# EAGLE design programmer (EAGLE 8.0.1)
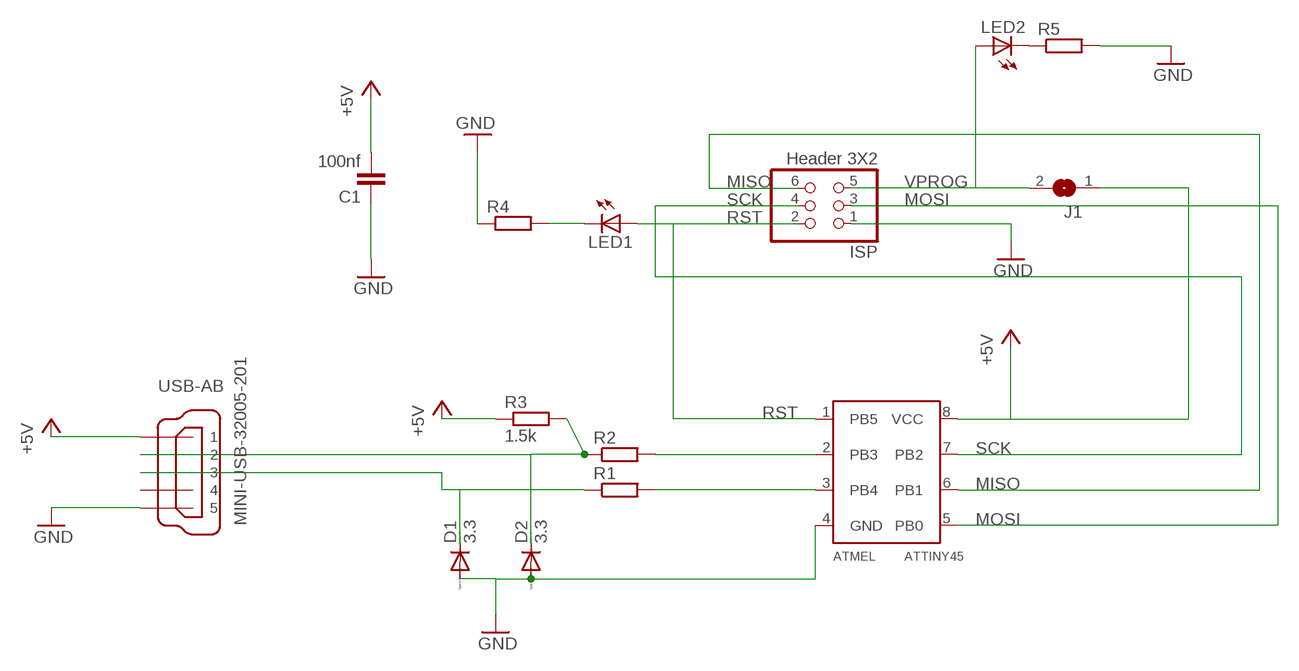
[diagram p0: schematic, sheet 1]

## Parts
ATMEL  ATTINY45  [SOIC8]
C1  100nf  C-EUC1206  [C1206]
D1  3.3  DIODE-MINIMELF  [MINIMELF]
D2  3.3  DIODE-MINIMELF  [MINIMELF]
ISP  Header 3X2  PINHD-2X3SMT  [2X03_SMT]
J1  SJW  [SJW]
LED1  LEDSMT1206  [1206]
LED2  LEDSMT1206  [1206]
R1  R-EU_R1206  [R1206]
R2  R-EU_R1206  [R1206]
R3  1.5k  R-EU_R1206  [R1206]
R4  R-EU_R1206  [R1206]
R5  R-EU_R1206  [R1206]
USB-AB  MINI-USB-32005-201  [32005-201]

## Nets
+5V: ATMEL.8(VCC) C1.2 J1.1 R3.1 USB-AB.1
GND: ATMEL.4(GND) C1.1 D1.A D2.A ISP.1 R4.1 R5.2 USB-AB.5
MISO: ATMEL.6(PB1) ISP.6
MOSI: ATMEL.5(PB0) ISP.3
N$1: ATMEL.2(PB3) R2.2
N$2: ATMEL.3(PB4) R1.2
N$3: LED2.C R5.1
N$4: LED1.C R4.2
N$5: D2.C R2.1 R3.2 USB-AB.2
N$6: D1.C R1.1 USB-AB.3
RST: ATMEL.1(PB5) ISP.2 LED1.A
SCK: ATMEL.7(PB2) ISP.4
VPROG: ISP.5 J1.2 LED2.A
Unconnected: USB-AB.4

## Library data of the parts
ATMEL = attiny45:ATTINY45
C1 = rcl:C-EU: CAPACITOR, European symbol
D1 D2 = diode:DIODE-: DIODE
ISP = pinhead+:PINHD-2X3: PIN HEADER
J1 = jumper:SJ: SMD solder JUMPER
LED1 LED2 = led:LED: LED
R1-R5 = rcl:R-EU_: RESISTOR, European symbol
USB-AB = con-cypressindustries:MINI-USB-: MINI USB-B Conector Source: www.cypressindustries.com; OC_FARNELL: unknown; OC_NEWARK: unknown

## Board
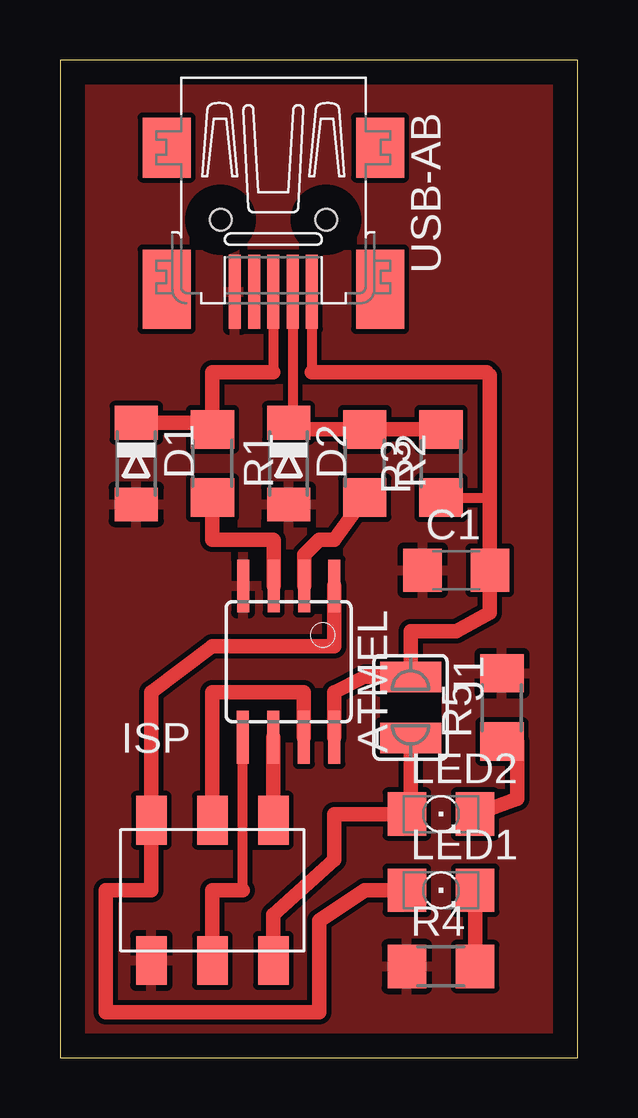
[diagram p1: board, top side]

Size 21.57 x 41.58 mm. Coordinates in mm from the lower left corner, seen from the top.
Outline: 0,0 21.57,0 21.57,41.58 0,41.58 0,0
Copper layers (1*16): Top 0.035mm / dielectric 1.5mm / Bottom 0.035mm
Design rules "default": minimum track width 10mil, minimum drill 24mil, track to track 8mil, track to pad 8mil, pad to pad 8mil, via to via 8mil, smd to smd 8mil, copper to edge 40mil, drill to drill 8mil, minimum pad ring 10mil, minimum via ring 8mil, stop-mask expansion 4mil, vias tented up to drill 0mil, thermal gap 10mil
tRestrict: area 13.3,14 to 15.9,15.2

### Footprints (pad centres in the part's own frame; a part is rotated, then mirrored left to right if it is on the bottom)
SOIC8 = smd 0.5 x 2.2: 1 -1.905,-3.154; 2 -0.645,-3.154; 3 0.625,-3.154; 4 1.895,-3.154; 5 1.905,3.154; 6 0.635,3.154; 7 -0.635,3.154; 8 -1.905,3.154
C1206 = smd 1.6 x 1.8: 1 -1.4,0; 2 1.4,0
MINIMELF = smd 1.4 x 1.8: A 1.7,0; C -1.7,0
2X03_SMT = smd 1.27 x 2.032: 1 -2.54,-2.921; 2 -2.54,2.921; 3 0,-2.921; 4 0,2.921; 5 2.54,-2.921; 6 2.54,2.921
SJW = smd 1.27 x 2.54: 1 -1.27,0; 2 1.27,0
1206 = smd 1.6 x 1.803: A -1.422,0; C 1.422,0
R1206 = smd 1.6 x 1.803: 1 -1.422,0; 2 1.422,0
32005-201 = smd 3.1 x 0.5: 1 3,1.6; 2 3,0.8; 3 3,0; 4 3,-0.8; 5 3,-1.6 | smd 2.5 x 2: M1 -3,-4.45; M2 -3,4.45 | smd 3.3 x 2: M3 2.9,4.45; M4 2.9,-4.45 | hole 0.9: 0,2.2; 0,-2.2

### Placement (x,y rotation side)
ATMEL  9.53,16.51 180 top
C1  16.51,20.32 0 top
D1  3.17,24.77 270 top
D2  9.53,24.77 270 top
ISP  6.35,6.98 0 top
J1  14.6,14.6 270 top
LED1  15.87,6.98 0 top
LED2  15.87,10.16 0 top
R1  6.35,24.77 270 top
R2  12.7,24.77 270 top
R3  15.87,24.77 90 top
R4  15.87,3.81 0 top
R5  18.41,14.6 90 top
USB-AB  8.89,34.92 270 top

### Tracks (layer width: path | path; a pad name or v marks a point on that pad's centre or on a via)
+5V
  Top 0.406: 17.78,28.57 17.91,28.44 | USB-AB.1 10.49,28.57 | R3.1 17.91,23.34 17.91,23.49
  Top 0.61: ATMEL.8 11.43,15.24 12.7,15.88 J1.1 14.6,17.78 16.51,17.78 17.91,18.54 C1.2 17.91,23.49 17.91,28.44 | 10.49,28.57 17.78,28.57
GND
  pour Top: 0,42.54 21.59,42.54 21.59,-1.27 0,-1.27
MISO
  Top 0.61: ISP.6 ATMEL.6
MOSI
  Top 0.406: 7.62,6.98 ATMEL.5
  Top 0.61: ISP.3 6.35,6.98 7.62,6.98
N$1
  Top 0.61: ATMEL.2 10.17,20.96 10.79,21.59 11.43,21.59 R2.2
N$2
  Top 0.406: 8.9,21.58 8.89,21.59
  Top 0.61: ATMEL.3 8.9,21.58 | 8.89,21.59 6.35,21.59 R1.2
N$3
  Top 0.406: 19.05,13.18 R5.1
  Top 0.61: LED2.C 19.05,10.79 19.05,13.18
N$4
  Top 0.406: LED1.C 17.27,7.62
  Top 0.61: R4.2 LED1.C
N$5
  Top 0.406: USB-AB.2 9.69,26.46 D2.C 9.53,26.19
  Top 0.61: R3.2 R2.1 9.53,26.19
N$6
  Top 0.406: USB-AB.3 8.89,28.57 | R1.1 6.35,26.46
  Top 0.61: 8.89,28.57 6.35,28.57 R1.1 | 6.35,26.46 D1.C
RST
  Top 0.61: LED1.A 12.7,6.98 10.79,5.71 10.79,1.9 1.9,1.9 1.9,6.98 3.81,6.98 ISP.2 3.81,15.24 6.35,17.14 11.43,17.14 ATMEL.1
SCK
  Top 0.61: ISP.4 6.35,15.24 10.16,15.24 ATMEL.7
VPROG
  Top 0.406: LED2.A 14.6,10.79
  Top 0.61: ISP.5 8.89,5.97 11.43,8.25 11.43,10.16 LED2.A | 14.6,10.79 J1.2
